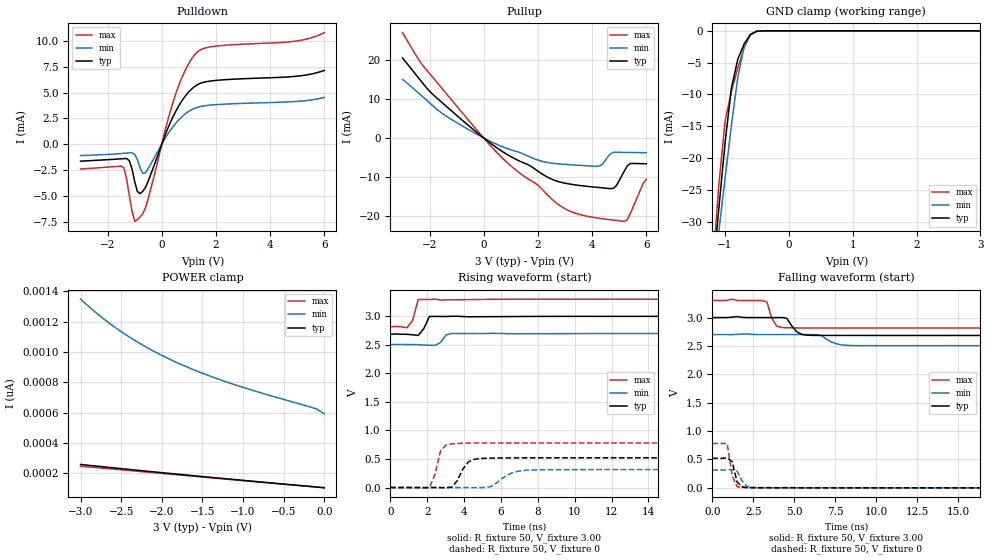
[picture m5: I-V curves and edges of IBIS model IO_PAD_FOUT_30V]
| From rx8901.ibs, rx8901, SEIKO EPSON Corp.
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[Model]   IO_PAD_FOUT_30V
Model_type 3-state
Enable Active-High
Polarity Non-Inverting
Vmeas=1.50
C_comp   2.5p   2.0p   3.0p
[Temperature Range] 25   105   -40
[Voltage Range]   3.00   2.70   3.30
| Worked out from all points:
|   slope of the pulldown table from 0 to 0.45 V, typ, clamps not added: 158 ohm
|   slope of the pullup table from 0 to 0.45 V, typ, clamps not added: 193 ohm
|   GND clamp passes 1 mA (typ) near -0.63 V on its own axis
|   falling waveform, R_fixture 50, V_fixture 3.00: 20-80 % time 492ps typ, 749ps min, 388ps max; typ from 3 V to 2.69 V
|   falling waveform, R_fixture 50, V_fixture 0: 20-80 % time 263ps typ, 410ps min, 312ps max; typ from 0.521 V to 0 V
|   rising waveform, R_fixture 50, V_fixture 3.00: 20-80 % time 310ps typ, 264ps min, 266ps max; typ from 2.69 V to 3 V
|   rising waveform, R_fixture 50, V_fixture 0: 20-80 % time 574ps typ, 892ps min, 385ps max; typ from 0 V to 0.521 V
[Pullup]
-3V       20.45mA    14.99mA    26.95mA
-2.4V     15.29mA    11.46mA    20.02mA
-1.9V     11.29mA    8.359mA    15.65mA
300mV     -1.589mA   -1.035mA   -2.327mA
1.2V      -5.477mA   -3.426mA   -8.267mA
2V        -8.47mA    -5.635mA   -12.03mA
2.9V      -11.4mA    -6.67mA    -17.67mA
4.2V      -12.61mA   -7.222mA   -20.45mA
4.8V      -12.81mA   -3.651mA   -20.96mA
5.2V      -8.293mA   -3.68mA    -21.28mA
5.4V      -6.536mA   -3.697mA   -19.5mA
6V        -6.57mA    -3.748mA   -10.6mA
[Pulldown]
-3V       -1.645mA   -1.105mA   -2.404mA
-1.4V     -1.401mA   -881.9uA   -2.281mA
-1.2V     -1.594mA   -838.2uA   -4.933mA
-1V       -3.61mA    -971.9uA   -7.472mA
-800mV    -4.793mA   -2.307mA   -7.046mA
-600mV    -4.172mA   -2.75mA    -6.158mA
500mV     3.112mA    1.977mA    4.757mA
900mV     4.773mA    3.003mA    7.349mA
1.3V      5.744mA    3.563mA    8.902mA
2V        6.182mA    3.832mA    9.508mA
5V        6.596mA    4.15mA     10.01mA
6V        7.149mA    4.527mA    10.82mA
[GND Clamp]
-3V       -252mA     -211.1mA   -302.4mA
-1.2V     -38.9mA    -40.17mA   -37.89mA
-1.1V     -28.19mA   -31.69mA   -24.51mA
-1V       -17.59mA   -23.23mA   -14.19mA
-900mV    -8.971mA   -14.82mA   -9.505mA
-800mV    -4.446mA   -7.29mA    -5.815mA
-700mV    -2.032mA   -2.407mA   -2.638mA
-600mV    -545.5uA   -567.8uA   -606uA
-500mV    -57.02uA   -91.22uA   -35.65uA
3V        103.3pA    656.8pA    92.53pA
[POWER Clamp]
-3V       257.8pA    1.349nA    246.5pA
-2.8V     246.6pA    1.255nA    236.9pA
-2.7V     241.1pA    1.212nA    232.1pA
-2.5V     230.2pA    1.134nA    222.5pA
-2.2V     214.2pA    1.035nA    208.2pA
-1.9V     198.5pA    951.5pA    193.9pA
-1.6V     183.1pA    881.1pA    179.6pA
-1.3V     167.9pA    820.4pA    165.3pA
-800mV    143pA      733.7pA    141.6pA
-100mV    108.6pA    625.2pA    109.9pA
0V        103.3pA    592.3pA    105.6pA
[Falling Waveform]
R_fixture=50
V_fixture=3.00
V_fixture_min=2.70
V_fixture_max=3.30
0s        3V         2.7V       3.3V
3.333ns   3V         2.7V       3.275V
3.636ns   3V         2.7V       2.983V
3.939ns   3V         2.7V       2.85V
4.242ns   3V         2.7V       2.825V
4.545ns   2.987V     2.7V       2.82V
5.152ns   2.748V     2.7V       2.818V
6.061ns   2.687V     2.7V       2.817V
8.485ns   2.685V     2.508V     2.817V
30ns      2.685V     2.505V     2.817V
[Falling Waveform]
R_fixture=50
V_fixture=0
V_fixture_min=0
V_fixture_max=0
0s        521.3mV    314.6mV    782mV
606.1ps   520.1mV    313.8mV    781mV
909.1ps   527.5mV    313.7mV    780.5mV
1.212ns   461.8mV    323.3mV    215.5mV
1.515ns   101.8mV    295.3mV    21.12mV
1.818ns   17.94mV    124.1mV    7.129mV
2.121ns   6.284mV    23.69mV    4.666mV
2.424ns   3.428mV    9.908mV    3.696mV
3.03ns    1.964mV    2.907mV    2.613mV
30ns      20.71uV    21.68uV    25.37uV
[Rising Waveform]
R_fixture=50
V_fixture=3.00
V_fixture_min=2.70
V_fixture_max=3.30
0s        2.685V     2.505V     2.816V
909.1ps   2.685V     2.506V     2.801V
1.212ns   2.677V     2.505V     2.93V
1.515ns   2.665V     2.504V     3.296V
1.818ns   2.785V     2.498V     3.296V
2.121ns   2.998V     2.492V     3.295V
2.727ns   2.998V     2.542V     3.287V
3.03ns    2.997V     2.677V     3.289V
3.333ns   3.001V     2.699V     3.291V
30ns      3V         2.7V       3.3V
[Rising Waveform]
R_fixture=50
V_fixture=0
V_fixture_min=0
V_fixture_max=0
0s        2.167nV    4.547nV    2.013nV
2.121ns   -1.402mV   97.81uV    -821uV
2.424ns   -48.27uV   -233.4uV   231.1mV
2.727ns   -556.1uV   -2.15mV    647mV
3.333ns   8.321mV    -232uV     765.3mV
4.242ns   449.8mV    -298.1uV   778mV
4.848ns   507.4mV    -1.408mV   780.4mV
6.667ns   519.6mV    265mV      781.5mV
7.576ns   520.5mV    305.5mV    781.7mV
30ns      521.3mV    314.5mV    782mV
[Ramp]
R_load=50
dV/dt_r   3.128E-1/5.237E-10   1.887E-1/8.578E-10   4.692E-1/3.202E-10
dV/dt_f   1.891E-1/4.653E-10   1.172E-1/7.303E-10   2.901E-1/3.198E-10
|[End   IO_PAD_FOUT_30V
